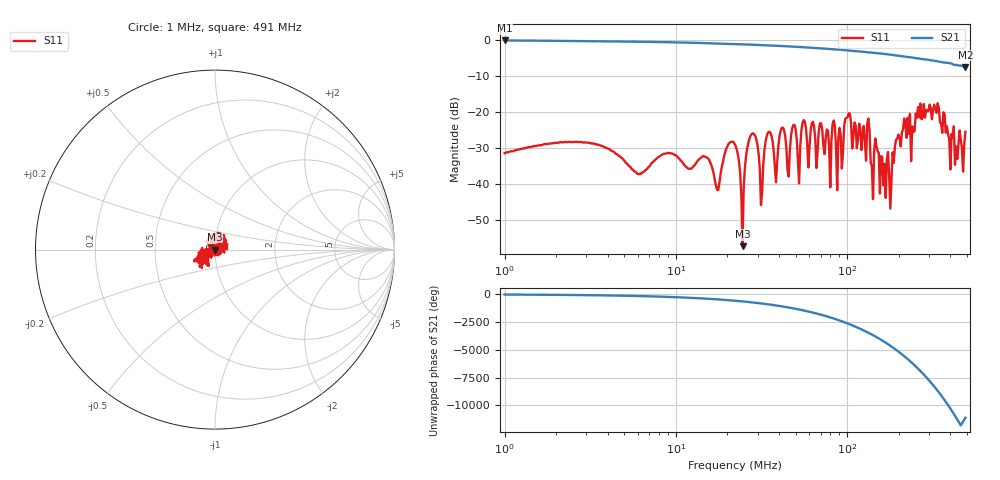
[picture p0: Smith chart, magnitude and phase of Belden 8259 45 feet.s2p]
! ListType=Log
!!Belden 8259 45 feet
# MHZ S RI R 50
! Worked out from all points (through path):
!   400 points, 1 MHz to 491 MHz, reference 50 ohm
!   highest |S21| = -0.19 dB at 1 MHz (marker M1); lowest = -7.5 dB at 491 MHz (marker M2)
!   lowest |S11| = -57.2 dB at 24.51 MHz (marker M3), VSWR 1.00, Z = 49.9 - j0.092 ohm
!   |S11| at or under -10 dB: start of sweep to end of sweep
!   S12 and S22 are empty: the file has one direction only
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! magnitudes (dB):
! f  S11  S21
! 1 MHz  -31.4  -0.2
! 2.831 MHz  -28.4  -0.4
! 8.013 MHz  -32.4  -0.6
! 22.33 MHz  -29.4  -1.2
! 24.51 MHz  -57.2  -1.3
! 27.33 MHz  -26.6  -1.4
! 31.43 MHz  -45.8  -1.5
! 34.5 MHz  -25.8  -1.6
! 38.46 MHz  -39.5  -1.7
! 49.3 MHz  -23.6  -1.9
! 52.46 MHz  -39.8  -2.0
! 62.24 MHz  -23.1  -2.2
! 77.35 MHz  -25.2  -2.5
! 79.79 MHz  -40.9  -2.6
! 82.31 MHz  -23.4  -2.6
! 87.59 MHz  -41.7  -2.7
! 102.3 MHz  -20.4  -3.0
! 133.2 MHz  -21.8  -3.5
! 141.7 MHz  -44.2  -3.6
! 176.2 MHz  -37.7  -4.1
! 267.9 MHz  -17.7  -5.3
! 491 MHz  -25.5  -7.5
